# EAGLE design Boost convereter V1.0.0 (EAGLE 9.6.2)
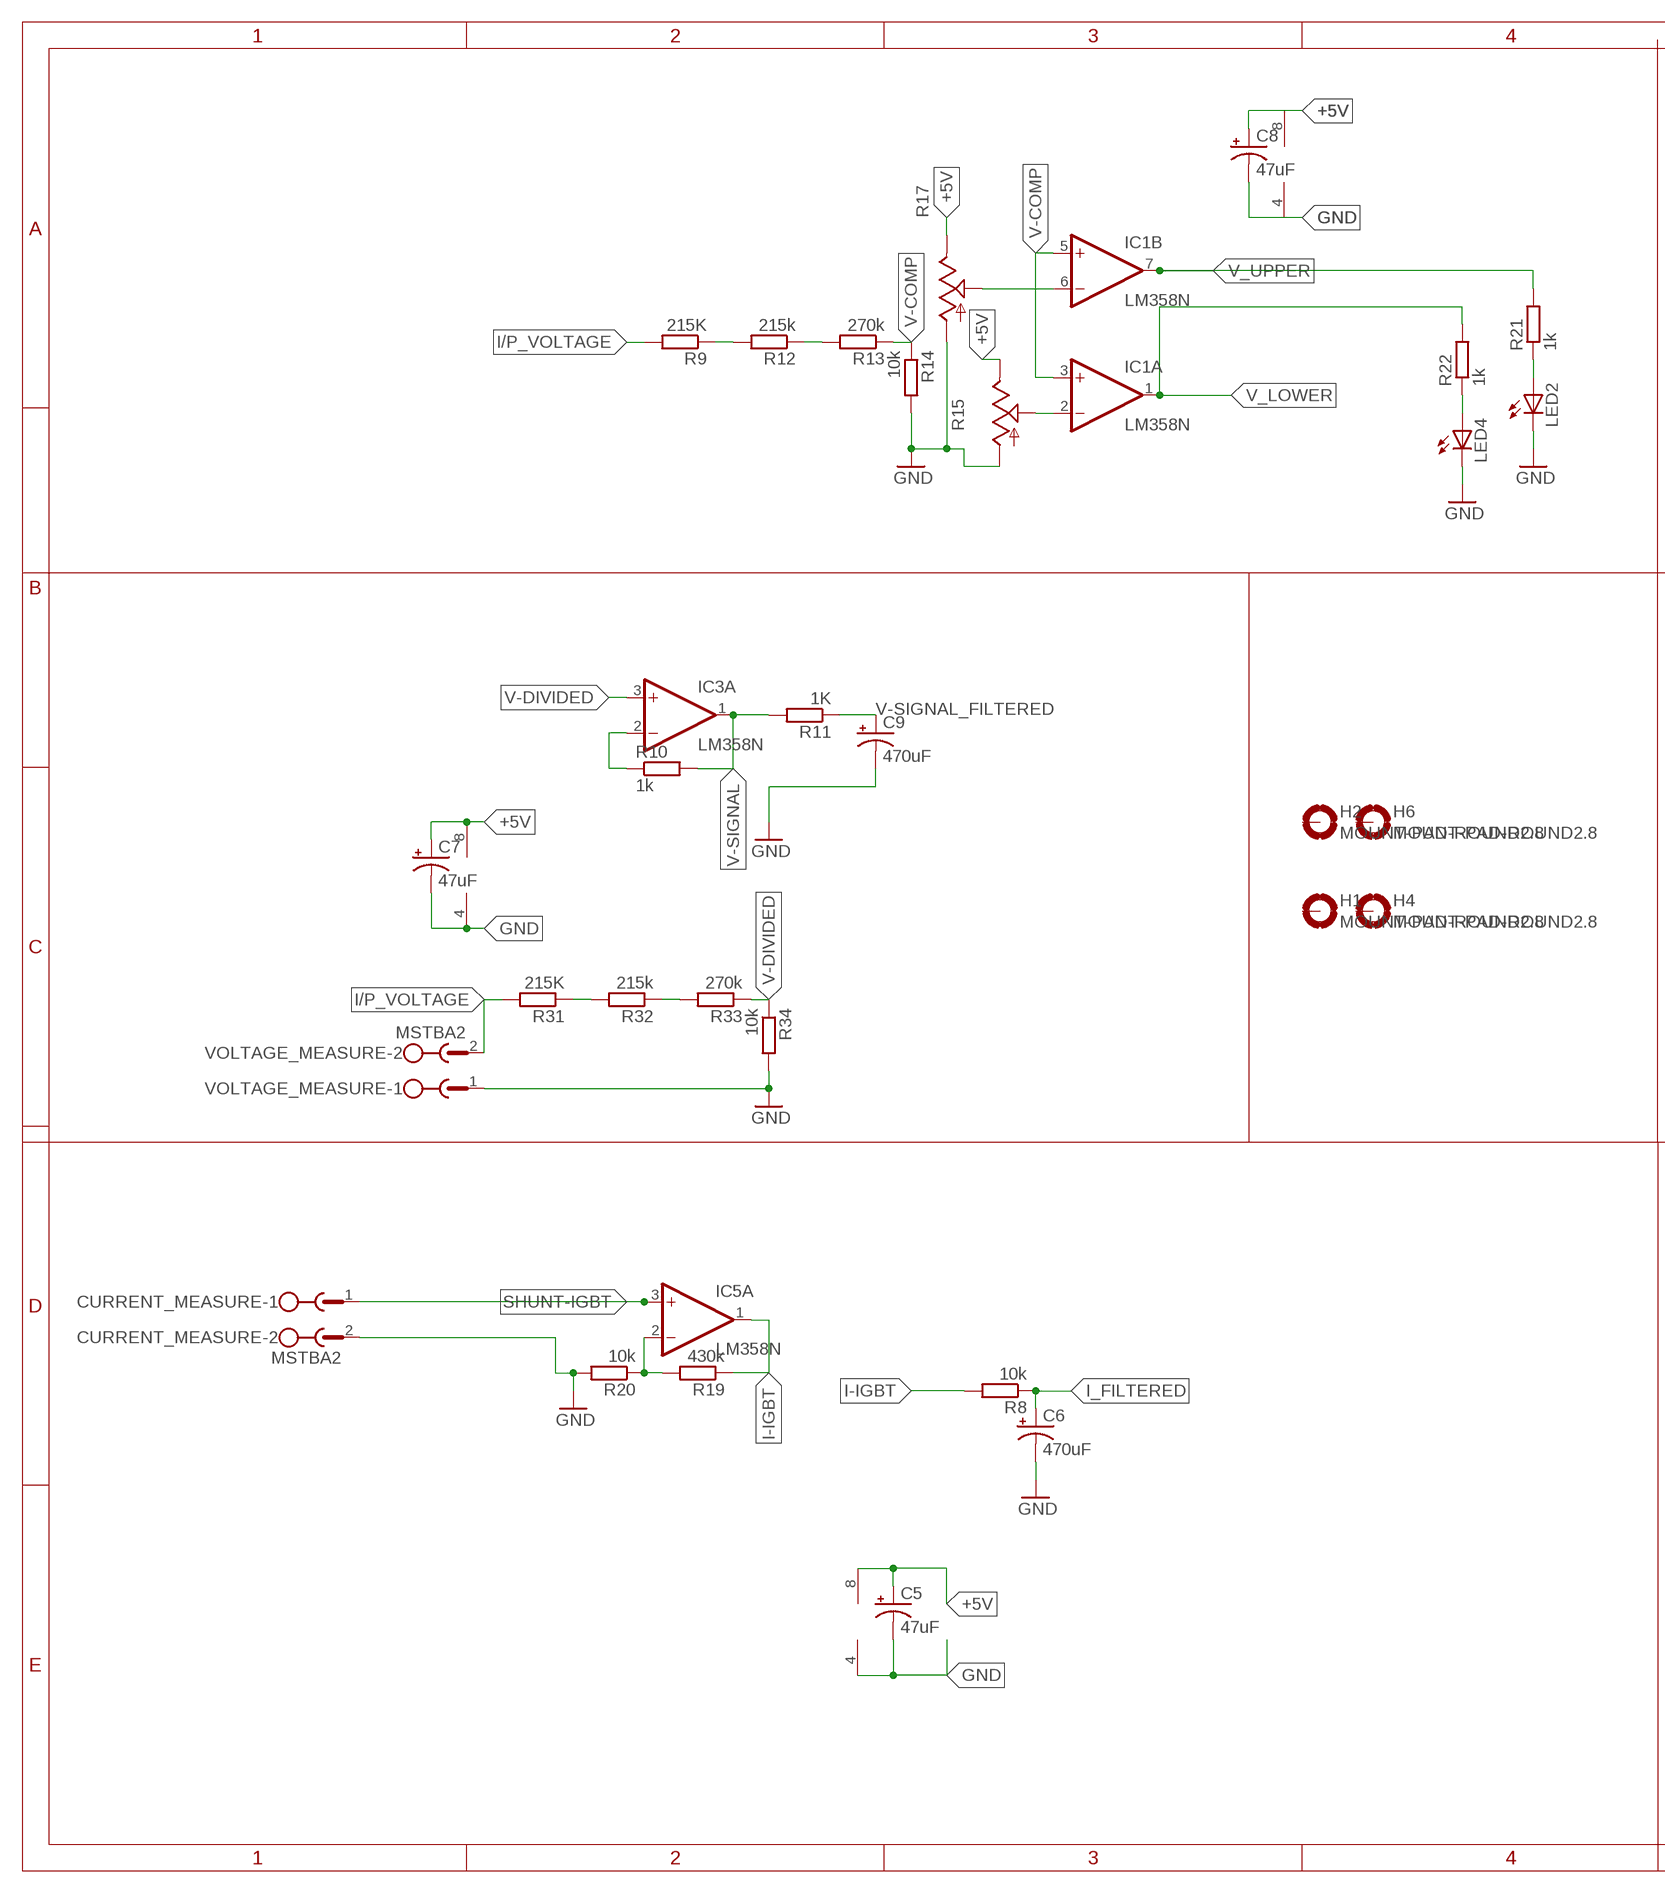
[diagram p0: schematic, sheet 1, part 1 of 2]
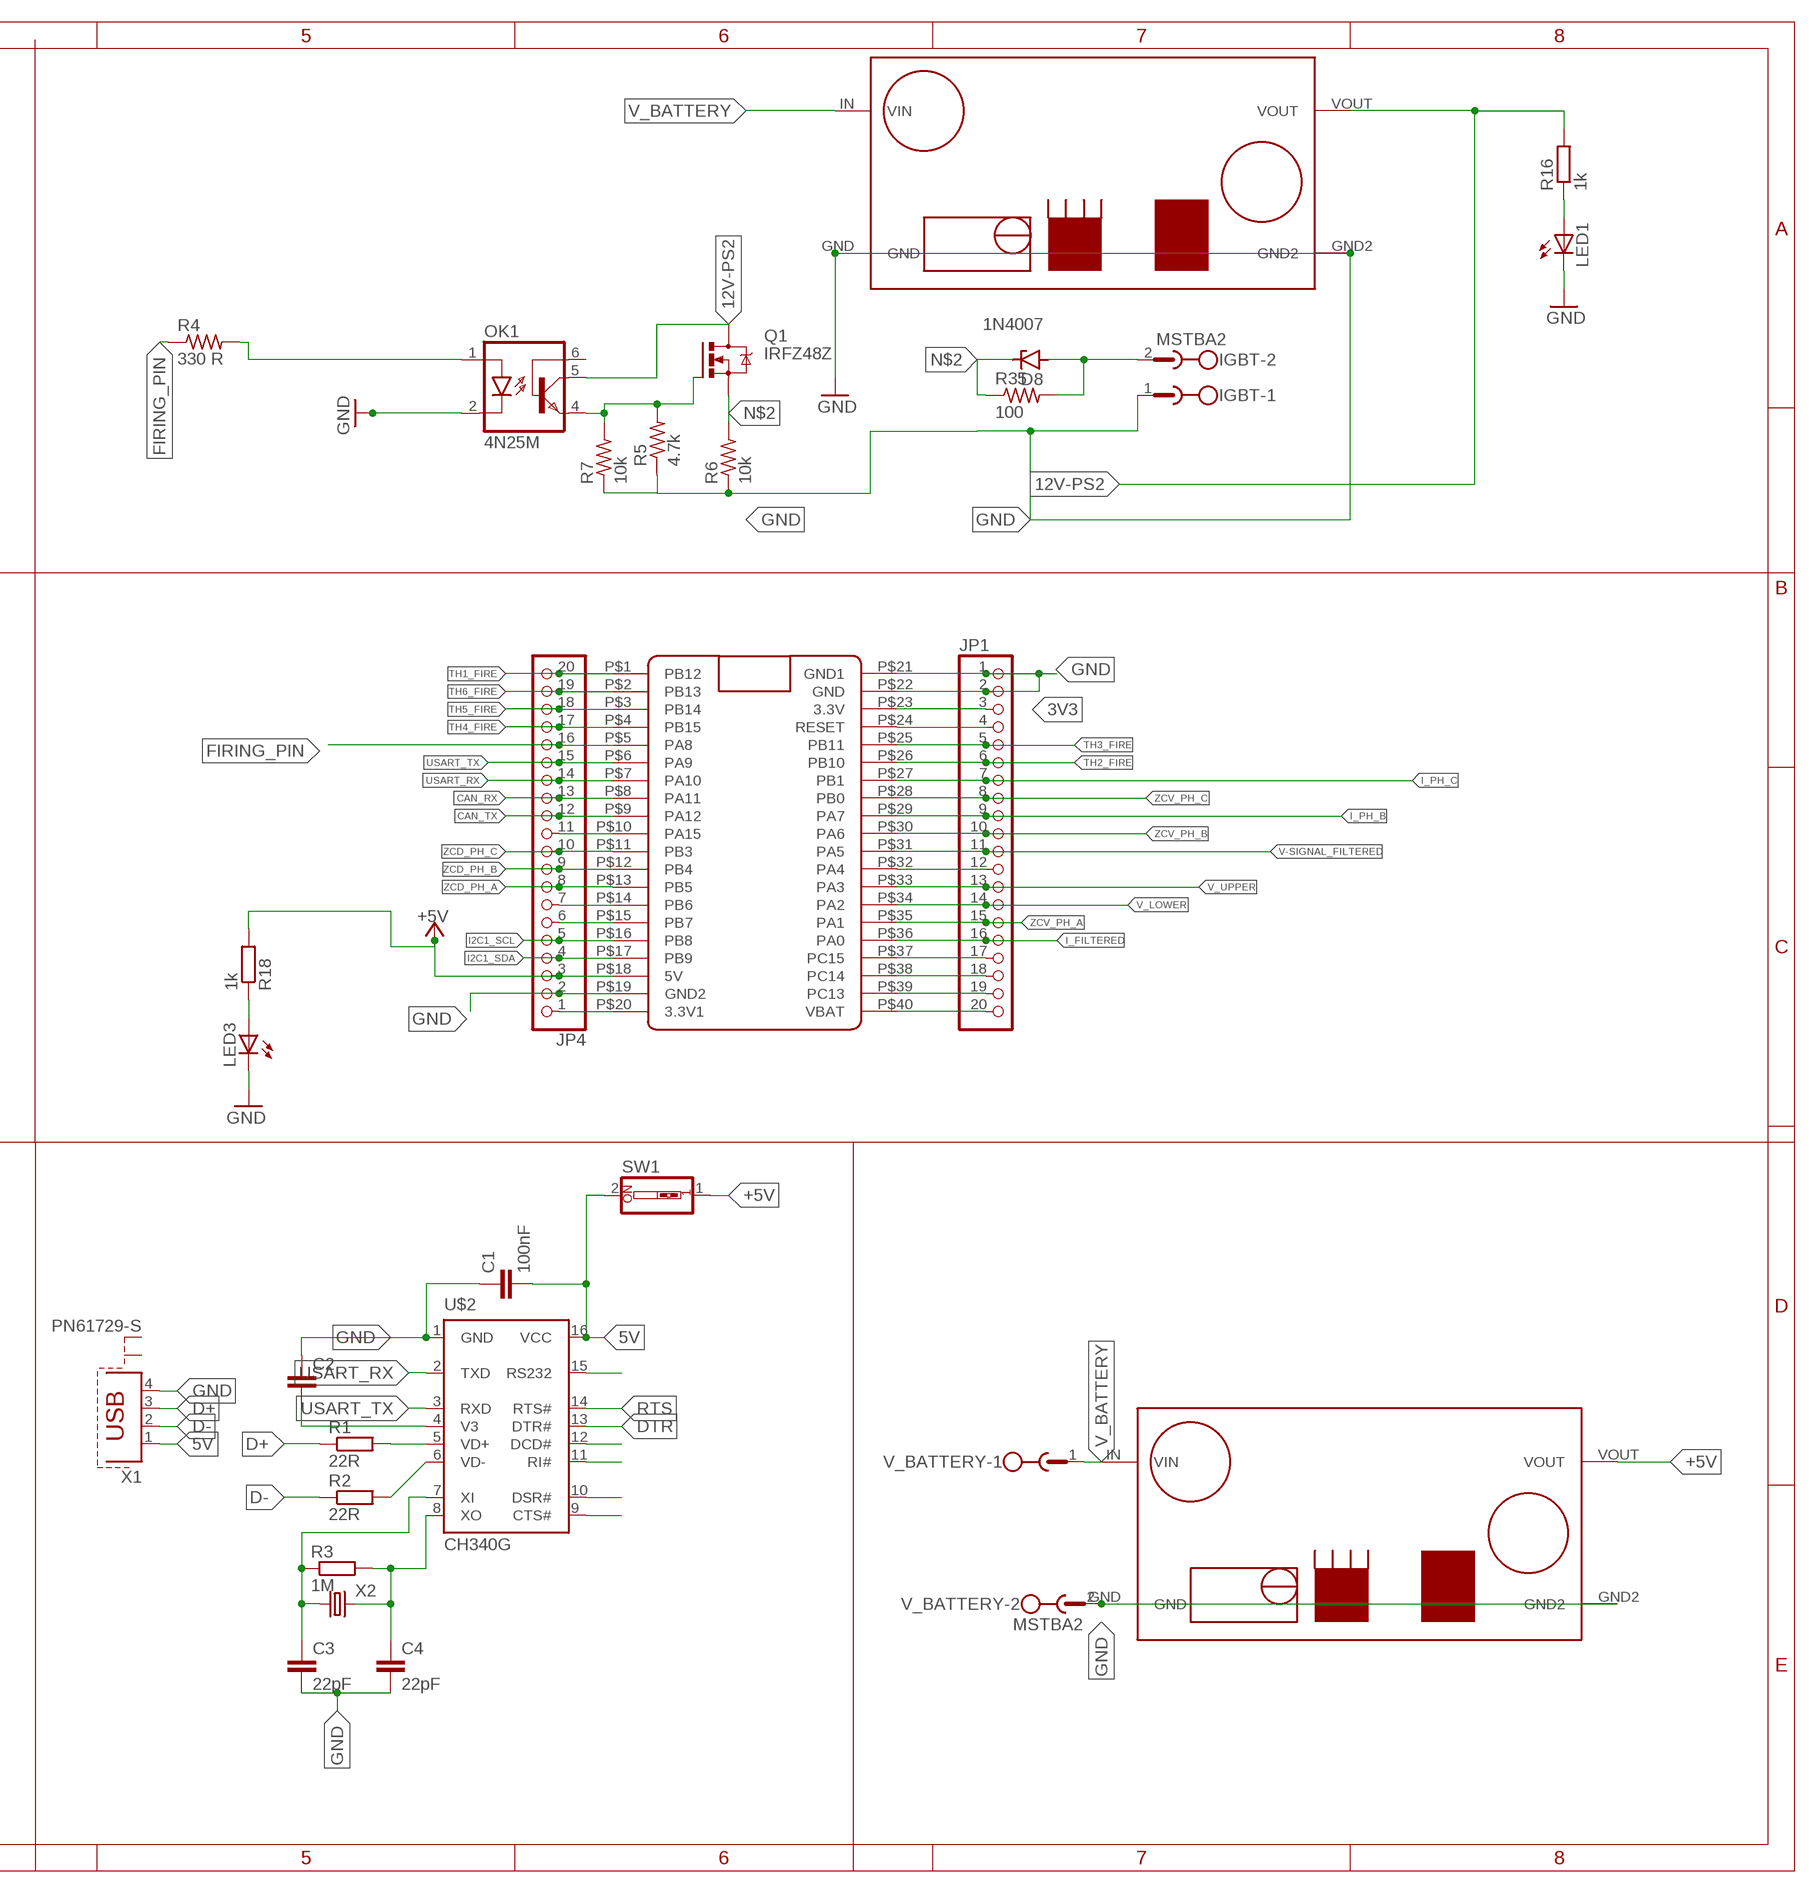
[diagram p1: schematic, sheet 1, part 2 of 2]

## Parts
C1  100nF  C2,5-3  [C2.5-3]
C2  C2,5-3  [C2.5-3]
C3  22pF  C2,5-3  [C2.5-3]
C4  22pF  C2,5-3  [C2.5-3]
C5  47uF  CPOL-USE3.5-8  [E3,5-8]
C6  470uF  CPOL-USE3.5-8  [E3,5-8]
C7  47uF  CPOL-USE3.5-8  [E3,5-8]
C8  47uF  CPOL-USE3.5-8  [E3,5-8]
C9  470uF  CPOL-USE3.5-8  [E3,5-8]
CURRENT_MEASURE  MSTBA2  [MSTBA2]
D8  1N4007  1N821  [DO35Z10]
H1  MOUNT-PAD-ROUND2.8  [2,8-PAD]
H2  MOUNT-PAD-ROUND2.8  [2,8-PAD]
H4  MOUNT-PAD-ROUND2.8  [2,8-PAD]
H6  MOUNT-PAD-ROUND2.8  [2,8-PAD]
IC1  LM358N  [DIL08]
IC3  LM358N  [DIL08]
IC5  LM358N  [DIL08]
IGBT  MSTBA2  [MSTBA2]
JP1  PINHD-1X20  [1X20]
JP4  PINHD-1X20  [1X20]
LED1  LEDB156  [Q62902-B156]
LED2  LEDB156  [Q62902-B156]
LED3  LEDB156  [Q62902-B156]
LED4  LEDB156  [Q62902-B156]
OK1  4N25M  [DIL06]
Q1  IRFZ48Z  [TO220BH]
R1  22R  R-EU_0207/7  [0207/7]
R2  22R  R-EU_0207/7  [0207/7]
R3  1M  R-EU_0207/7  [0207/7]
R4  330 R  R-US_0207/10  [0207/10@2]
R5  4.7k  R-US_0207/10  [0207/10@2]
R6  10k  R-US_0207/10  [0207/10@2]
R7  10k  R-US_0207/10  [0207/10@2]
R8  10k  R-EU_0207/10  [0207/10]
R9  215K  R-EU_0207/10  [0207/10]
R10  1k  R-EU_0207/10  [0207/10]
R11  1K  R-EU_0207/10  [0207/10]
R12  215k  R-EU_0207/10  [0207/10]
R13  270k  R-EU_0207/10  [0207/10]
R14  10k  R-EU_0207/10  [0207/10]
R15  TRIM_US-RJ9W  [RJ9W]
R16  1k  R-EU_0207/10  [0207/10]
R17  TRIM_US-RJ9W  [RJ9W]
R18  1k  R-EU_0207/10  [0207/10]
R19  430k  R-EU_0207/10  [0207/10]
R20  10k  R-EU_0207/10  [0207/10]
R21  1k  R-EU_0207/10  [0207/10]
R22  1k  R-EU_0207/10  [0207/10]
R31  215K  R-EU_0207/10  [0207/10]
R32  215k  R-EU_0207/10  [0207/10]
R33  270k  R-EU_0207/10  [0207/10]
R34  10k  R-EU_0207/10  [0207/10]
R35  100  R-US_0207/10  [0207/10@2]
SW1  SW_DIP-1  [EDG-01]
U$1  BLUE_PILL  [BLUE_PILL]
U$2  CH340G  [CH340]
U$3  XL7015  [XL7015]
U$4  XL7015  [XL7015]
V_BATTERY  MSTBA2  [MSTBA2]
VOLTAGE_MEASURE  MSTBA2  [MSTBA2]
X1  PN61729-S  [PN61729-S]
X2  CRYSTALS-NOGND-HC49/4H  [HC49]

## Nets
3V3: JP1.3 U$1.P$23(3.3V)
5V: C1.2 SW1.2 U$2.16(VCC) X1.1
12V-PS2: OK1.5(COL) Q1.D R16.2 U$4.VOUT
+5V: C5.+ C7.+ C8.+ IC1.8(P:V+) IC3.8(P:V+) IC5.8(P:V+) JP4.3 R15.E R17.E R18.2 SW1.1 U$1.P$18(5V) U$3.VOUT
CAN_RX: JP4.13 U$1.P$8(PA11)
CAN_TX: JP4.12 U$1.P$9(PA12)
D+: R1.1 X1.3
D-: R2.1 X1.2
DTR: U$2.13(DTR#)
FIRING_PIN: JP4.16 R4.1 U$1.P$5(PA8)
GND: C1.1 C2.1 C3.2 C4.2 C5.- C6.- C7.- C8.- C9.- CURRENT_MEASURE.2 IC1.4(P:V-) IC3.4(P:V-) IC5.4(P:V-) IGBT.1 JP1.1 JP1.2 JP4.2 LED1.K(C) LED2.K(C) LED3.K(C) LED4.K(C) OK1.2(C) R5.1 R6.1 R7.1 R14.2 R15.A R17.A R20.2 R34.2 U$1.P$19(GND2) U$1.P$21(GND1) U$1.P$22(GND) U$2.1(GND) U$3.GND U$3.GND2 U$4.GND U$4.GND2 V_BATTERY.2 VOLTAGE_MEASURE.1 X1.4
I2C1_SCL: JP4.5 U$1.P$16(PB8)
I2C1_SDA: JP4.4 U$1.P$17(PB9)
I-IGBT: IC5.1(A:OUT) R8.2 R19.1
I/P_VOLTAGE: R9.2 R31.2 VOLTAGE_MEASURE.2
I_FILTERED: C6.+ JP1.16 R8.1 U$1.P$36(PA0)
I_PH_B: JP1.9 U$1.P$29(PA7)
I_PH_C: JP1.7 U$1.P$27(PB1)
N$1: JP1.4 U$1.P$24(RESET)
N$2: D8.C Q1.S R6.2 R35.1
N$3: R1.2 U$2.5(VD+)
N$4: R2.2 U$2.6(VD-)
N$5: JP1.12 U$1.P$32(PA4)
N$6: U$2.15(RS232)
N$7: U$2.12(DCD#)
N$8: U$2.11(RI#)
N$9: U$2.10(DSR#)
N$10: U$2.9(CTS#)
N$11: C3.1 R3.1 U$2.7(XI) X2.1
N$12: C4.1 R3.2 U$2.8(XO) X2.2
N$13: OK1.1(A) R4.2
N$14: OK1.4(EMI) Q1.G R5.2 R7.2
N$15: R9.1 R12.2
N$16: IC5.2(A:-IN) R19.2 R20.1
N$17: JP1.17 U$1.P$37(PC15)
N$18: JP1.18 U$1.P$38(PC14)
N$19: JP1.19 U$1.P$39(PC13)
N$20: JP1.20 U$1.P$40(VBAT)
N$21: JP4.1 U$1.P$20(3.3V1)
N$22: R31.1 R32.2
N$23: R32.1 R33.2
N$24: IC3.2(A:-IN) R10.1
N$25: R12.1 R13.2
N$26: JP4.6 U$1.P$15(PB7)
N$27: JP4.7 U$1.P$14(PB6)
N$28: IC1.2(A:-IN) R15.S
N$29: IC1.6(B:-IN) R17.S
N$30: LED2.A R21.1
N$31: JP4.11 U$1.P$10(PA15)
N$32: LED1.A R16.1
N$33: D8.A IGBT.2 R35.2
N$34: LED3.A R18.1
N$35: LED4.A R22.1
N$2222: C2.2 U$2.4(V3)
RTS: U$2.14(RTS#)
SHUNT-IGBT: CURRENT_MEASURE.1 IC5.3(A:+IN)
TH1_FIRE: JP4.20 U$1.P$1(PB12)
TH2_FIRE: JP1.6 U$1.P$26(PB10)
TH3_FIRE: JP1.5 U$1.P$25(PB11)
TH4_FIRE: JP4.17 U$1.P$4(PB15)
TH5_FIRE: JP4.18 U$1.P$3(PB14)
TH6_FIRE: JP4.19 U$1.P$2(PB13)
USART_RX: JP4.14 U$1.P$7(PA10) U$2.2(TXD)
USART_TX: JP4.15 U$1.P$6(PA9) U$2.3(RXD)
V-COMP: IC1.3(A:+IN) IC1.5(B:+IN) R13.1 R14.1
V-DIVIDED: IC3.3(A:+IN) R33.1 R34.1
V-SIGNAL: IC3.1(A:OUT) R10.2 R11.2
V-SIGNAL_FILTERED: C9.+ JP1.11 R11.1 U$1.P$31(PA5)
V_BATTERY: U$3.IN(VIN) U$4.IN(VIN) V_BATTERY.1
V_LOWER: IC1.1(A:OUT) JP1.14 R22.2 U$1.P$34(PA2)
V_UPPER: IC1.7(B:OUT) JP1.13 R21.2 U$1.P$33(PA3)
ZCD_PH_A: JP4.8 U$1.P$13(PB5)
ZCD_PH_B: JP4.9 U$1.P$12(PB4)
ZCD_PH_C: JP4.10 U$1.P$11(PB3)
ZCV_PH_A: JP1.15 U$1.P$35(PA1)
ZCV_PH_B: JP1.10 U$1.P$30(PA6)
ZCV_PH_C: JP1.8 U$1.P$28(PB0)
Unconnected: H1.B2,8(MOUNT) H2.B2,8(MOUNT) H4.B2,8(MOUNT) H6.B2,8(MOUNT) IC3.5(B:+IN) IC3.6(B:-IN) IC3.7(B:OUT) IC5.5(B:+IN) IC5.6(B:-IN) IC5.7(B:OUT) OK1.6(BAS) X1.S1 X1.S2

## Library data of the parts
C1-C4 = capacitor-wima:C: CAPACITOR
C5-C9 = rcl:CPOL-US: POLARIZED CAPACITOR, American symbol; SPICEPREFIX: C
CURRENT_MEASURE IGBT V_BATTERY VOLTAGE_MEASURE = con-phoenix-508:MSTBA2: PHOENIX; MF: FARNELL; MPN: 1757242; OC_FARNELL: 3705171; OC_NEWARK: 71C4161
D8 = diode:1N821: Reference DIODE
H1 H2 H4 H6 = holes:MOUNT-PAD-ROUND: MOUNTING PAD, round
IC1 IC3 IC5 = linear:LM358: OP AMP also LM158; LM258; LM2904 Source: http://cache.national.com/ds/LM/LM158.pdf
JP1 JP4 = pinhead:PINHD-1X20: PIN HEADER
LED1-LED4 = led:LED: LED
OK1 = optocoupler:4N*?M: General Purpose 6-Pin Phototransistor Optocouplers Source: http://www.fairchildsemi.com/ds/4N/4N35-M.pdf; MPN: 4N25-M; OC_FARNELL: 1021349; OC_NEWARK: 98K9084
Q1 = transistor-power:IRFZ48: N Channel HEXFET® Power MOSFET Logic Level Source: http://www.irf.com/product-info/datasheets/data/irfz48z.pdf
R1-R3 = resistor:R-EU_: RESISTOR, European symbol
R4-R7 R35 = rcl:R-US_: RESISTOR, American symbol; SPICEPREFIX: R
R8-R14 R16 R18-R22 R31-R34 = rcl:R-EU_: RESISTOR, European symbol; SPICEPREFIX: R
R15 R17 = pot:TRIM_US-: POTENTIOMETER
SW1 = special:SW_DIP-1: DIP SWITCH
U$1 = AP_BluePill:BLUE_PILL
U$2 = ch340G:CH340G
U$3 U$4 = xl7015:XL7015
X1 = con-berg:PN61729-S: BERG USB connector; OC_FARNELL: unknown; OC_NEWARK: unknown
X2 = IQD-Frequency-Products:CRYSTALS-NOGND: CRYSTALS CAN NOT GROUNDED

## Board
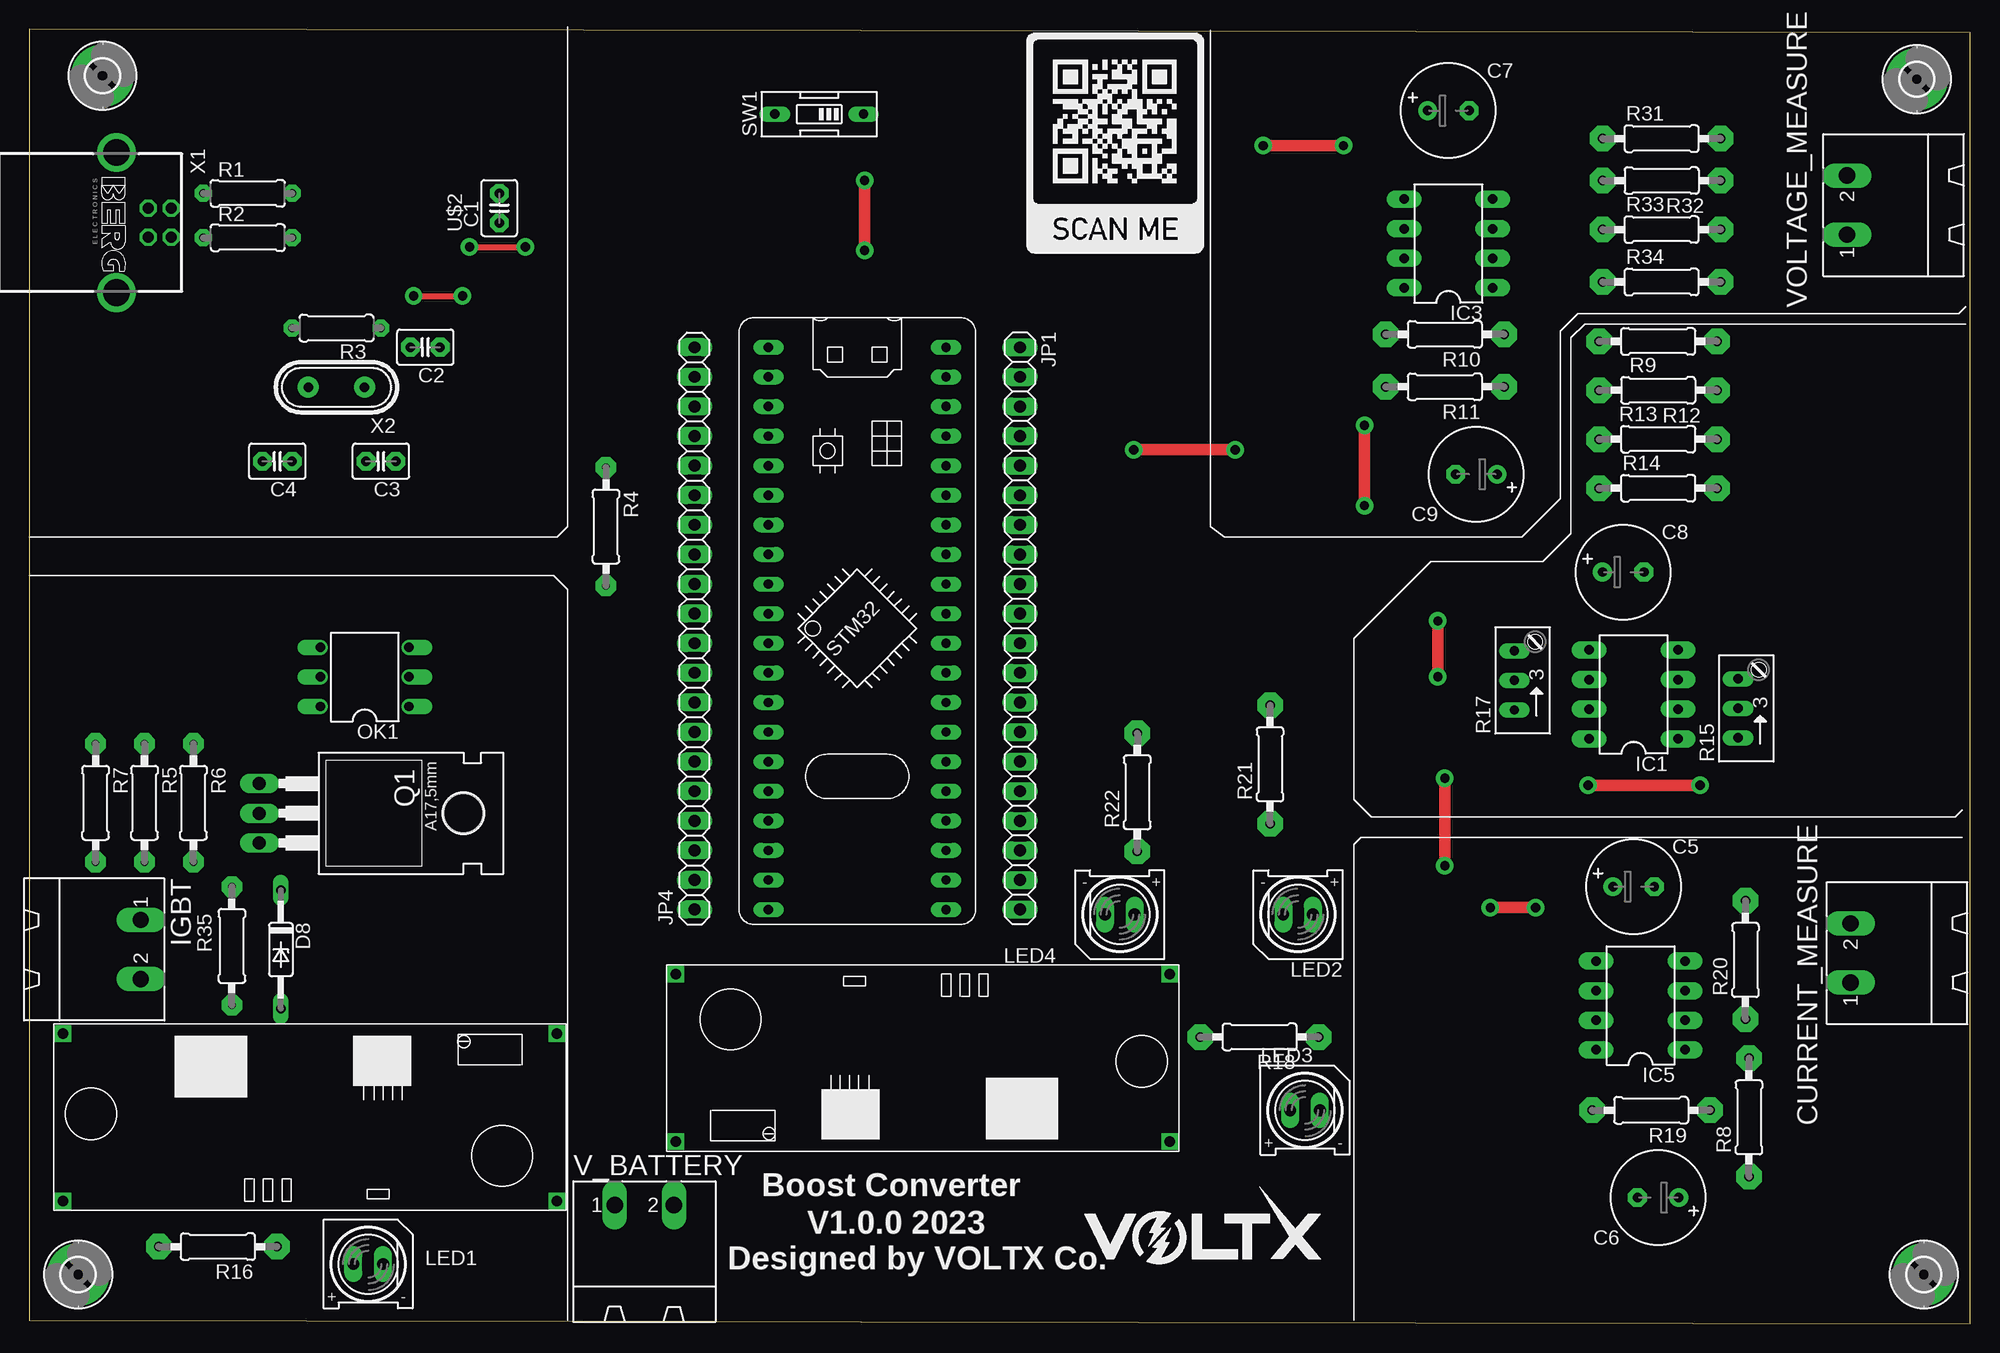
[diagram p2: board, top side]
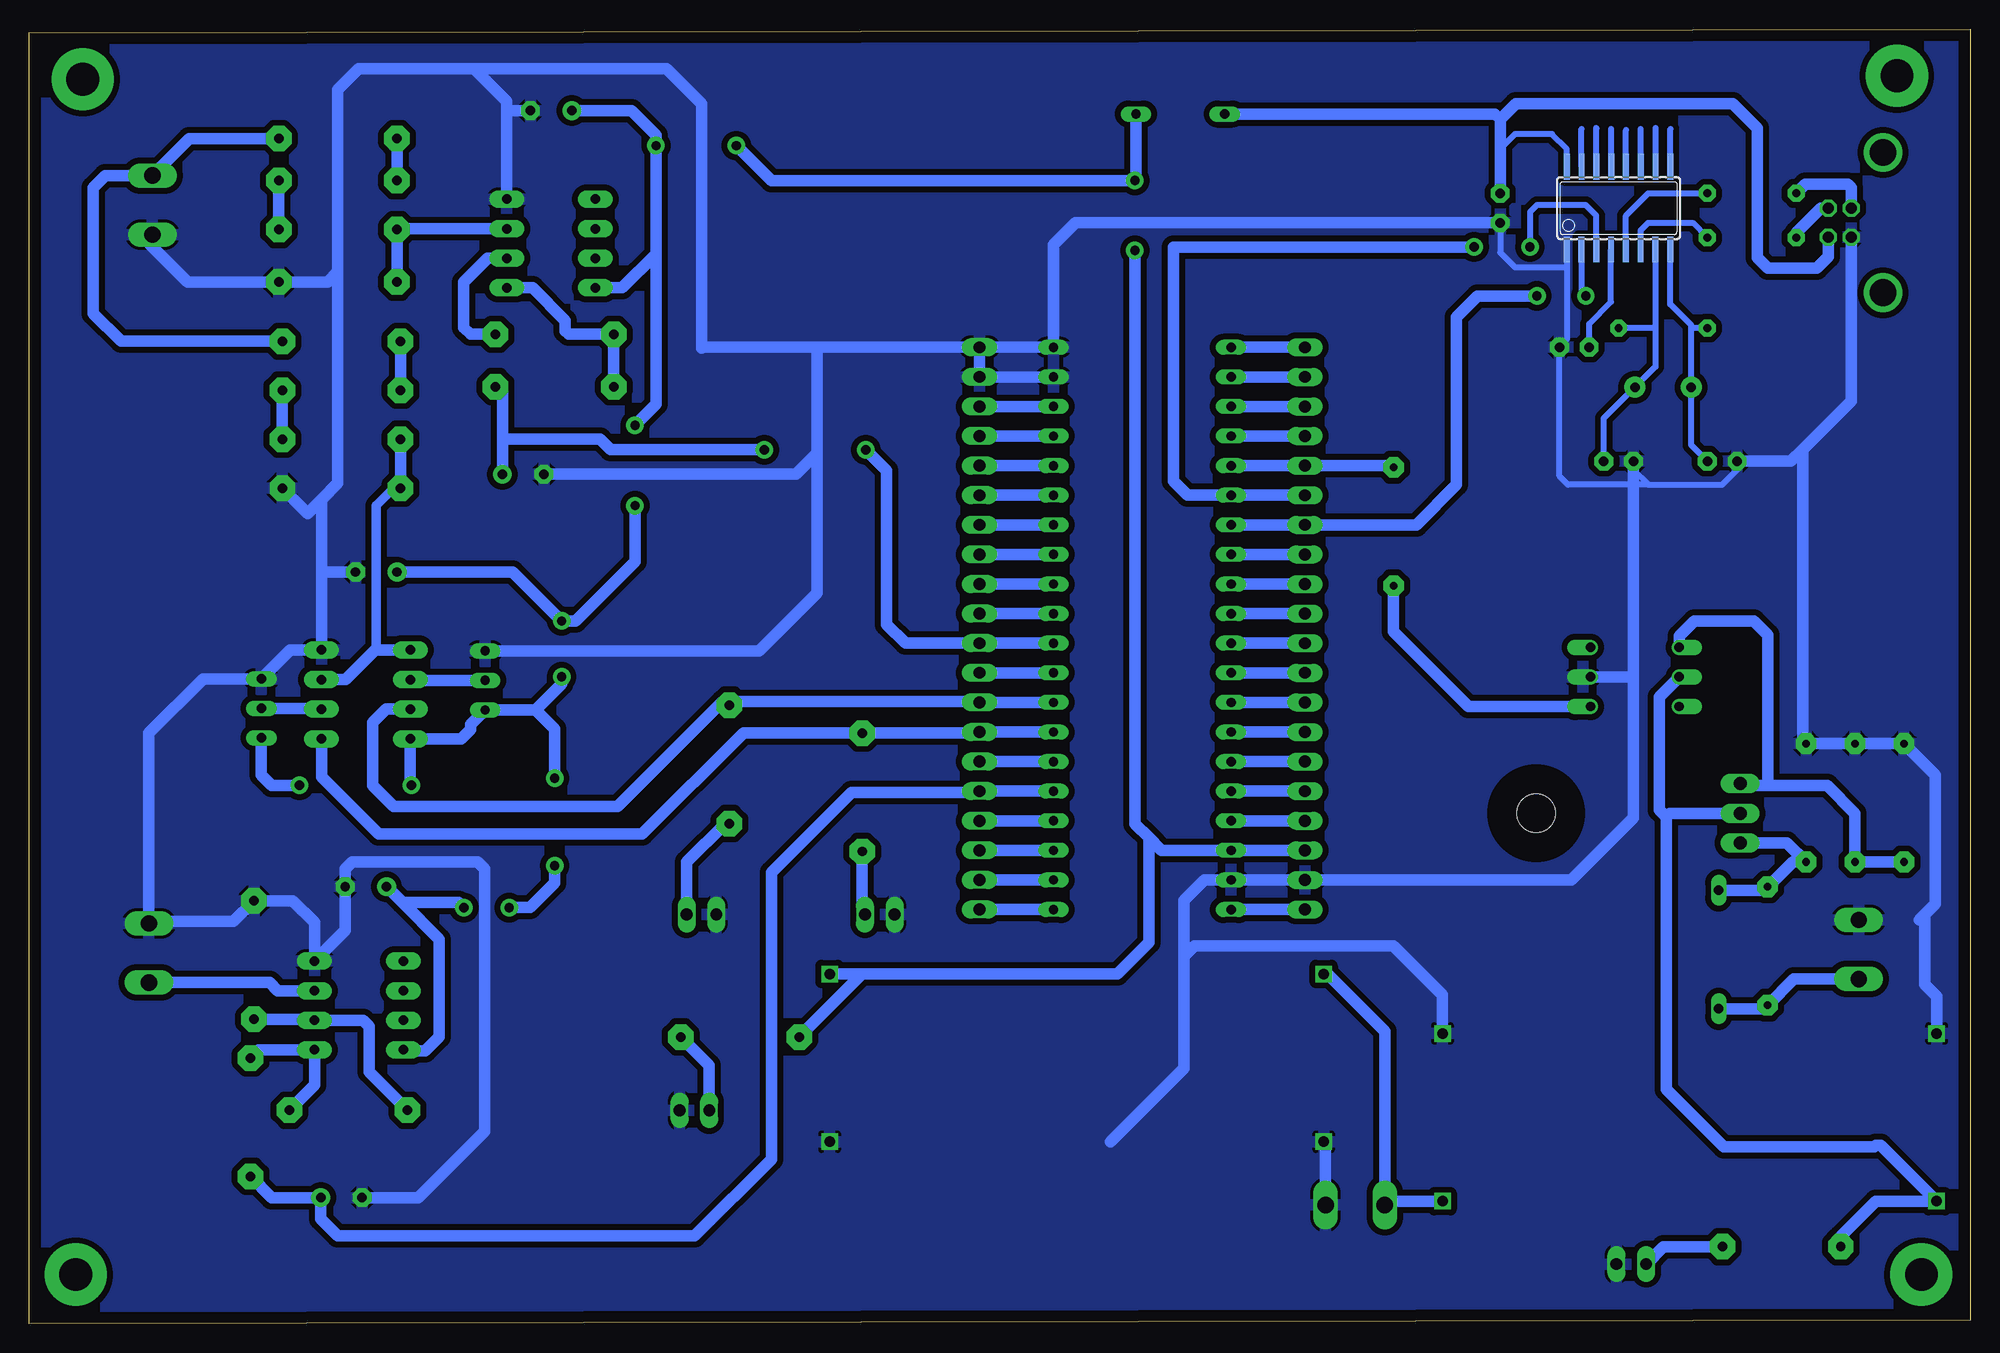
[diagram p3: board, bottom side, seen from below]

Size 166.6 x 111.1 mm. Coordinates in mm from the lower left corner, seen from the top.
Outline: 0,0.3 166.6,0 166.6,110.8 0,111.1 0,0.3
Copper layers (1*16): Top 0.035mm / dielectric 1.5mm / Bottom 0.035mm
Design rules "default *": minimum track width 6mil, minimum drill 0.35mm, track to track 20mil, track to pad 20mil, pad to pad 6mil, via to via 6mil, smd to smd 6mil, copper to edge 40mil, drill to drill 6mil, minimum pad ring 10mil, minimum via ring 8mil, stop-mask expansion 4mil, vias tented up to drill 0mil, thermal gap 10mil

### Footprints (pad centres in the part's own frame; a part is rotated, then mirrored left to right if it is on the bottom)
C2.5-3 = drill 0.813 pad 1.6 octagon: 1 -1.27,0; 2 1.27,0
E3,5-8 = drill 0.813 pad 1.6: + -1.778,0 | drill 0.813 pad 1.6 octagon: - 1.778,0
MSTBA2 = drill 1.397 long: 1 -2.54,5.08; 2 2.54,5.08
DO35Z10 = drill 0.813 long: A 5.08,0; C -5.08,0
2,8-PAD = drill 2.8 pad 5.334: B2,8 0,0
DIL08 = drill 0.813 pad 1.5 long: 1 -3.81,-3.81; 2 -1.27,-3.81; 3 1.27,-3.81; 4 3.81,-3.81; 5 3.81,3.81; 6 1.27,3.81; 7 -1.27,3.81; 8 -3.81,3.81
1X20 = drill 1.016 long: 1 -24.13,0; 2 -21.59,0; 3 -19.05,0; 4 -16.51,0; 5 -13.97,0; 6 -11.43,0; 7 -8.89,0; 8 -6.35,0; 9 -3.81,0; 10 -1.27,0; 11 1.27,0; 12 3.81,0; 13 6.35,0; 14 8.89,0; 15 11.43,0; 16 13.97,0; 17 16.51,0; 18 19.05,0; 19 21.59,0; 20 24.13,0
Q62902-B156 = drill 1.016 long: A -1.27,0; K 1.27,0
DIL06 = drill 0.813 offset: 1 -2.54,-3.81; 2 0,-3.81; 3 2.54,-3.81; 4 2.54,3.81; 5 0,3.81; 6 -2.54,3.81
TO220BH = drill 1.118 long: D 0,-6.35; G -2.54,-6.35; S 2.54,-6.35 | hole 3.302: 0,11.176
0207/7 = drill 0.686 pad 1.448 octagon: 1 -3.81,0; 2 3.81,0
0207/10@2 = drill 0.65 pad 1.778 octagon: 1 -5.08,0; 2 5.08,0
0207/10 = drill 0.813 pad 2.184 octagon: 1 -5.08,0; 2 5.08,0
RJ9W = drill 0.813 long: A 2.54,0.635; E -2.54,0.635; S 0,0.635
EDG-01 = drill 0.813 long: 1 0,-3.81; 2 0,3.81
BLUE_PILL = drill 0.8 long: P$1 -7.62,15.24; P$2 -7.62,12.7; P$3 -7.62,10.16; P$4 -7.62,7.62; P$5 -7.62,5.08; P$6 -7.62,2.54; P$7 -7.62,0; P$8 -7.62,-2.54; P$9 -7.62,-5.08; P$10 -7.62,-7.62; P$11 -7.62,-10.16; P$12 -7.62,-12.7; P$13 -7.62,-15.24; P$14 -7.62,-17.78; P$15 -7.62,-20.32; P$16 -7.62,-22.86; P$17 -7.62,-25.4; P$18 -7.62,-27.94; P$19 -7.62,-30.48; P$20 -7.62,-33.02; P$21 7.62,15.24; P$22 7.62,12.7; P$23 7.62,10.16; P$24 7.62,7.62; P$25 7.62,5.08; P$26 7.62,2.54; P$27 7.62,0; P$28 7.62,-2.54; P$29 7.62,-5.08; P$30 7.62,-7.62; P$31 7.62,-10.16; P$32 7.62,-12.7; P$33 7.62,-15.24; P$34 7.62,-17.78; P$35 7.62,-20.32; P$36 7.62,-22.86; P$37 7.62,-25.4; P$38 7.62,-27.94; P$39 7.62,-30.48; P$40 7.62,-33.02
CH340 = smd 0.5 x 2.2: 1 -4.445,-3.55; 2 -3.185,-3.55; 3 -1.915,-3.55; 4 -0.645,-3.55; 5 0.635,-3.55; 6 1.895,-3.55; 7 3.165,-3.55; 8 4.435,-3.55; 9 4.445,3.55; 10 3.175,3.55; 11 1.905,3.55; 12 0.635,3.55; 13 -0.635,3.55; 14 -1.905,3.55; 15 -3.175,3.55; 16 -4.445,3.55
XL7015 = drill 0.9 square: GND -11.1,-5.1; GND2 31.3,-5.1; IN -11.1,9.3; VOUT 31.3,9.3
PN61729-S = drill 0.95 octagon: 1 1.25,4.71; 2 -1.25,4.71; 3 -1.25,2.71; 4 1.25,2.71 | drill 2.3 pad 2.9: S1 -6.02,0; S2 6.02,0
HC49 = drill 0.813 pad 1.8: 1 -2.413,0; 2 2.413,0

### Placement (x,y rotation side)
C1  40.35,95.74 90 top
C2  34,83.8 180 top
C3  30.19,74.01 180 top
C4  21.3,74.01 180 top
C5  137.7,37.5 0 top
C6  139.8,10.8 180 top
C7  121.8,104.1 0 top
C8  136.8,64.5 0 top
C9  124.2,72.9 180 top
CURRENT_MEASURE  161.4,31.8 90 top
D8  21.6,32.1 270 top
H1  162,106.8 0 top
H2  162.6,4.2 0 top
H4  6.3,107.1 0 top
H6  4.2,4.2 0 top
IC1  137.7,54 90 top
IC3  121.8,92.7 90 top
IC5  138.3,27.3 90 top
IGBT  4.5,32.1 270 top
JP1  85.04,59.66 270 top
JP4  57.1,59.66 90 top
LED1  29.1,5.1 0 top
LED2  108.9,35.1 180 top
LED3  109.5,18.3 0 top
LED4  93.6,35.1 180 top
OK1  28.8,55.5 90 top
Q1  26.1,43.8 270 top
R1  18.76,97.01 0 top
R2  18.76,93.2 0 top
R3  26.38,85.44 180 top
R4  49.5,68.4 270 top
R5  9.9,44.7 270 top
R6  14.1,44.7 270 top
R7  5.7,44.7 270 top
R8  147.6,17.7 90 top
R9  139.8,84.3 0 top
R10  121.5,84.9 180 top
R11  121.5,80.4 180 top
R12  139.8,80.1 180 top
R13  139.8,75.9 0 top
R14  139.8,71.7 0 top
R15  147.3,52.8 90 top
R16  16.2,6.6 180 top
R17  128.1,55.2 90 top
R18  105.6,24.6 180 top
R19  139.2,18.3 180 top
R20  147.3,31.2 90 top
R21  106.5,48 90 top
R22  95.1,45.6 90 top
R31  140.1,101.7 0 top
R32  140.1,98.1 180 top
R33  140.1,93.9 0 top
R34  140.1,89.4 0 top
R35  17.4,32.4 270 top
SW1  67.8,103.8 90 top
U$1  71.07,68.55 0 top
U$2  30.19,95.74 0 bottom
U$3  66.6,20.7 0 top
U$4  34.2,19.8 180 top
U$8  [VOLTX_LOGO_0.8]  90.56,4.86 0 top
U$9  [SCAN2]  85.6,91.85 0 top
V_BATTERY  52.8,5.1 0 top
VOLTAGE_MEASURE  161.1,96 90 top
X1  7.5,94.5 270 top
X2  26.38,80.36 180 top

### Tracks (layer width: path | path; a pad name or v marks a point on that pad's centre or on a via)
3V3
  Bottom 1: JP1.3 U$1.P$23
5V
  Bottom 0.5: U$2.16 34.63,100.82 35.91,102.09 39.08,102.09 40.35,100.82 C1.2
  Bottom 1: C1.2 40.35,103.35 | 40.35,103.35 39,104.7 20.4,104.7 18.3,102.6 18.3,91.5 17.4,90.6 13.2,90.6 12.21,91.59 X1.1 | SW1.2 40.8,103.8 40.35,103.35
12V-PS2
  Bottom 1: 26.1,43.5 26.1,20.1 21.16,15.16 8.24,15.16 8.1,15.3 7.7,15.3 U$4.VOUT 8.1,10.5 11.12,7.48 R16.2 | 26.1,43.5 25.8,43.8 Q1.D 19.2,43.8 | OK1.5 26.7,53.79 26.7,44.1 26.1,43.5
+5V  (via drill 0.8 pad 1.5)
  Top 1: v71.7,98.1 v71.7,92.1 | v112.8,101.1 v105.9,101.1 | v120.9,55.5 v120.9,60.3 | v133.8,46.2 v143.4,46.2 | v114.6,70.2 v114.6,77.1 | v121.5,46.8 v121.5,39.3 | v125.4,35.7 v129.3,35.7
  Bottom 1: JP4.3 U$1.P$18 69.41,40.61 70.5,41.7 | v71.7,92.1 71.7,42.9 70.5,41.7 | C7.+ 114.9,104.1 112.8,102 v112.8,101.1 112.8,91.8 | IC3.8 115.71,88.89 112.8,91.8 | v105.9,101.1 102.9,98.1 v71.7,98.1 71.61,98.19 SW1.1 | 146.7,50.23 R15.E 146.67,47.06 145.8,46.2 v143.4,46.2 | C5.+ 134.56,36.14 | 134.56,36.14 131.4,32.98 131.4,24.6 132.6,23.4 134.4,23.4 IC5.8 | 123.14,52.66 R17.E 128.7,51.43 128.7,51 129.51,50.19 IC1.8 133.89,46.29 v133.8,46.2 | v120.9,55.5 120.9,54.9 123.14,52.66 | C8.+ 125.1,64.5 v120.9,60.3 119.7,60.3 114.6,65.4 v114.6,70.2 | v114.6,77.1 112.8,78.9 112.8,91.8 | 123.14,52.66 121.5,51.02 v121.5,46.8 | v121.5,39.3 121.5,37.8 123.6,35.7 v125.4,35.7 | v129.3,35.7 129.74,36.14 134.56,36.14 | U$3.VOUT 95.12,30 | 70.5,41.7 70.5,32.7 73.2,30 95.12,30 | R18.2 95.12,30
CAN_RX
  Bottom 1: JP4.13 U$1.P$8
CAN_TX
  Bottom 1: U$1.P$9 JP4.12
D+
  Bottom 1: R1.1 14.16,97.8 10.5,97.8 10.21,97.51 X1.3
D-
  Bottom 1: X1.2 12.85,95.75 14.95,93.65 R2.1
DTR
  Bottom 0.5: U$2.13 30.82,102.52
FIRING_PIN
  Bottom 1: U$1.P$5 JP4.16 49.65,73.63 R4.1
GND
  Bottom 0.5: U$2.1 34.63,90.66 | 34.63,90.66 34.63,84.43 C2.1 35.27,72.74 34.53,72 27.65,72 | C3.2 28.92,73.8 28.92,73.27 27.65,72 | 27.65,72 21.3,72 20.03,73.27 C4.2 | C1.1 40.35,91.93 39.08,90.66 34.63,90.66
  Bottom 1: X1.4 10.21,79.19 14.4,75 | C4.2 15.39,74.01 14.4,75 | JP1.1 U$1.P$21 78.69,92.58 76.8,94.47 C1.1 | JP1.2 84.9,81.25 | 84.9,81.25 U$1.P$22 | JP1.1 85.04,81.39 84.9,81.25 | 28.92,55.5 28.92,43.38 34.23,38.07 JP4.2 U$1.P$19 65.73,38.07 67.5,36.3 67.5,31.5 | 28.92,55.5 28.92,73.8 | OK1.2 28.92,55.5 | VOLTAGE_MEASURE.1 156.3,93.18 156.3,92.7 153,89.4 R34.2 141,89.4 140.1,90.3 | 125.61,104.1 125.61,104.91 128.4,107.7 | 125.61,104.1 IC3.4 | 140.1,90.3 140.1,105.9 138.3,107.7 128.4,107.7 | C7.- 125.61,104.1 | 128.4,107.7 111.9,107.7 108.9,104.7 108.9,83.7 108.81,83.79 99,83.79 | JP1.1 99,83.79 | 141.51,64.5 IC1.4 144.2,57.81 R15.A 151.66,55.34 156.32,50.68 CURRENT_MEASURE.2 156.74,34.34 156.9,34.5 149.08,34.5 R20.2 143.98,36.28 142.11,34.41 IC5.4 139.48,33.74 C5.- 139.48,39 138.88,39.6 128.1,39.6 127.5,39 127.5,16.5 133.2,10.8 C6.- | 141.51,64.5 141.51,70.73 | R14.2 142.71,69.53 141.51,70.73 | 140.1,90.3 140.1,72.14 141.51,70.73 | C8.- 141.51,64.5 | C9.- 100.8,72.9 99,74.7 | 99,74.7 99,83.79 | 99,74.7 99,62.7 103.96,57.74 R17.A | 67.5,31.5 67.5,21.9 73.8,15.6 | 3.92,35.1 3.92,29.1 2.9,28.08 U$4.GND2 | 4.38,34.64 3.92,35.1 | 3.92,35.1 3.02,36 3.02,47.1 R7.1 R5.1 R6.1 14.4,50.08 14.4,75 | U$4.GND 45.3,28.2 49.5,32.4 66.6,32.4 67.5,31.5 | V_BATTERY.2 55.34,15.44 U$3.GND
  pour Bottom: -0.3,111.6 165.6,111.6 166.5,110.7 166.5,0.3 0,0.3 0,111 -0.3,111.3
I2C1_SCL
  Bottom 1: U$1.P$16 JP4.5
I2C1_SDA
  Bottom 1: JP4.4 U$1.P$17
I-IGBT
  Bottom 1: R19.1 142.11,20.47 IC5.1 146.89,23.49 R8.2
I/P_VOLTAGE
  Bottom 1: R31.2 152.86,101.7 VOLTAGE_MEASURE.2 160.06,98.54 161.1,97.5 161.1,86.7 158.7,84.3 R9.2
I_FILTERED
  Bottom 1: R8.1 145.78,10.8 C6.+ 141.58,8.99 140.1,7.52 109.48,7.52 102.9,14.1 102.9,38.7 96,45.6 84.69,45.6 84.6,45.69 | U$1.P$36 84.6,45.69 | 84.6,45.69 JP1.16
I_PH_B
  Bottom 1: U$1.P$29 JP1.9
I_PH_C
  Bottom 1: JP1.7 U$1.P$27
N$1
  Bottom 1: U$1.P$24 JP1.4
N$2
  Bottom 1: Q1.S 15.74,41.26 R6.2 15.26,39.62 R35.1 17.7,37.18 D8.C
N$3
  Bottom 0.5: U$2.5 29.55,95.1 27.65,97.01 R1.2
N$4
  Bottom 0.5: R2.2 23.84,94.47 27.65,94.47 28.3,93.82 U$2.6
N$5
  Bottom 1: U$1.P$32 84.55,55.85 84.6,55.8 84.99,55.8 JP1.12
N$6
  Bottom 0.5: U$2.15 33.37,102.53
N$7
  Bottom 0.5: U$2.12 29.55,102.44
N$8
  Bottom 0.5: U$2.11 28.29,102.52
N$9
  Bottom 0.5: U$2.10 27.02,102.58 27,102.6
N$10
  Bottom 0.5: U$2.9 25.75,102.54
N$11
  Bottom 0.5: U$2.7 27.03,85.44 | 27.03,85.44 27.03,82.13 X2.1 31.46,77.69 C3.1 | 27.03,85.44 R3.1
N$12
  Bottom 0.5: 23.97,85.44 X2.2 23.97,75.41 C4.1 | 23.97,85.44 23.97,85.71 25.75,87.49 U$2.8 | R3.2 23.97,85.44
N$13
  Bottom 1: R4.2 49.5,59.4 43.06,52.96 OK1.1
N$14
  Bottom 1: 17.4,46.2 12.3,46.2 9.9,43.8 R5.2 R7.2 | 17.4,46.2 19.5,46.2 | 19.5,46.2 20.4,46.2 20.26,46.34 Q1.G | 19.06,46.64 19.5,46.2 | OK1.4 24.99,59.01 23.7,60.3 18.6,60.3 17.4,59.1 17.4,46.2
N$15
  Bottom 1: R12.2 R9.1
N$16
  Bottom 1: R20.1 142.2,26.12 IC5.2 137.93,26.03 137.4,25.5 137.4,21.58 R19.2
N$17
  Bottom 1: JP1.17 U$1.P$37
N$18
  Bottom 1: U$1.P$38 JP1.18
N$19
  Bottom 1: JP1.19 U$1.P$39
N$20
  Bottom 1: U$1.P$40 JP1.20
N$21
  Bottom 1: JP4.1 U$1.P$20
N$22
  Bottom 1: R32.2 135.02,100.82 135.3,101.1 135.3,101.42 R31.1
N$23
  Bottom 1: R32.1 R33.2
N$24
  Bottom 1: IC3.2 127.27,91.43 129.3,89.4 129.3,85.5 128.7,84.9 R10.1
N$25
  Bottom 1: R12.1 R13.2
N$26
  Bottom 1: JP4.6 U$1.P$15
N$27
  Bottom 1: U$1.P$14 JP4.7
N$28
  Bottom 1: IC1.2 141.58,52.8 R15.S
N$29
  Bottom 1: R17.S 133.82,55.2 IC1.6
N$30
  Bottom 1: LED2.A 110.17,39.6 106.85,42.92 R21.1
N$31
  Bottom 1: U$1.P$10 JP4.11
N$32
  Bottom 1: R16.1 26.33,6.6 LED1.A
N$33
  Bottom 1: D8.A 17.7,27.02 R35.2 15.16,29.56 IGBT.2
N$34
  Bottom 1: LED3.A 108.23,22.15 R18.1
N$35
  Bottom 1: LED4.A 95.1,35.33 R22.1
N$2222
  Bottom 0.5: C2.2 32.73,85.8 30.84,87.69 U$2.4
RTS
  Bottom 0.5: U$2.14 32.09,102.59 32.1,102.6
SHUNT-IGBT
  Bottom 1: CURRENT_MEASURE.1 145.96,29.26 145.27,28.57 IC5.3
TH1_FIRE
  Bottom 1: JP4.20 U$1.P$1 | U$1.P$1 64.11,83.79 64.2,83.7 63.54,83.7 U$1.P$1
TH2_FIRE
  Bottom 1: U$1.P$26 JP1.6
TH3_FIRE
  Bottom 1: JP1.5 U$1.P$25
TH4_FIRE
  Bottom 1: U$1.P$4 JP4.17
TH5_FIRE
  Bottom 1: JP4.18 U$1.P$3
TH6_FIRE
  Bottom 1: U$1.P$2 JP4.19
USART_RX  (via drill 0.8 pad 1.5)
  Top 0.5: v33,88.2 v37.2,88.2
  Bottom 0.5: U$2.2 33.38,88.57 v33,88.2
  Bottom 1: U$1.P$7 JP4.14 47.55,68.55 44.1,72 44.1,86.4 42.3,88.2 v37.2,88.2
USART_TX  (via drill 0.8 pad 1.5)
  Top 0.5: v37.8,92.4 v42.6,92.4
  Bottom 0.5: U$2.3 32.1,95.1 33,96 37.2,96 37.8,95.4 v37.8,92.4
  Bottom 1: JP4.15 U$1.P$6 67.19,71.09 68.4,72.3 68.4,92.4 v42.6,92.4
V-COMP
  Bottom 0.813: 136.8,57.9 136.8,70.2 135.3,71.7
  Bottom 1: R13.1 R14.1 135.3,71.7 | IC1.3 139.43,55.27 136.8,57.9 136.71,57.81 IC1.5
V-DIVIDED
  Bottom 1: R34.1 R33.1 134.95,93.97 IC3.3
V-SIGNAL
  Bottom 1: IC3.1 123.39,88.89 120.6,86.1 120.6,85.2 120.3,84.9 R10.2 R11.2
V-SIGNAL_FILTERED  (via drill 0.8 pad 1.5)
  Top 1: v103.5,75 v94.8,75
  Bottom 1: C9.+ 125.98,75.9 | 125.98,75.9 125.98,79.8 R11.1 | 125.98,75.9 117.6,75.9 116.7,75 v103.5,75 | v94.8,75 93,73.2 93,60 91.39,58.39 JP1.11 U$1.P$31
V_BATTERY
  Bottom 1: U$3.IN 55.2,30 50.26,25.06 V_BATTERY.1 49.94,10.5 U$4.IN
V_LOWER
  Bottom 1: IC1.1 141.51,46.89 136.62,42 114,42 105.3,50.7 95.12,50.7 | U$1.P$34 JP1.14 85.11,50.7 95.12,50.7 | R22.2 95.12,50.7
V_UPPER
  Bottom 1: U$1.P$33 JP1.13 85.13,53.4 106.82,53.4 | 106.82,53.4 107.1,53.4 116.1,44.4 135.3,44.4 137.1,46.2 137.1,51.6 135.97,52.73 IC1.7 | R21.2 106.82,53.4
ZCD_PH_A
  Bottom 1: JP4.8 U$1.P$13
ZCD_PH_B
  Bottom 1: U$1.P$12 JP4.9
ZCD_PH_C
  Bottom 1: JP4.10 U$1.P$11
ZCV_PH_A
  Bottom 1: JP1.15 U$1.P$35
ZCV_PH_B
  Bottom 1: JP1.10 U$1.P$30
ZCV_PH_C
  Bottom 1: U$1.P$28 JP1.8

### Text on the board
tPlace: Boost Converter | V1.0.0 2023 | Designed by VOLTX Co.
